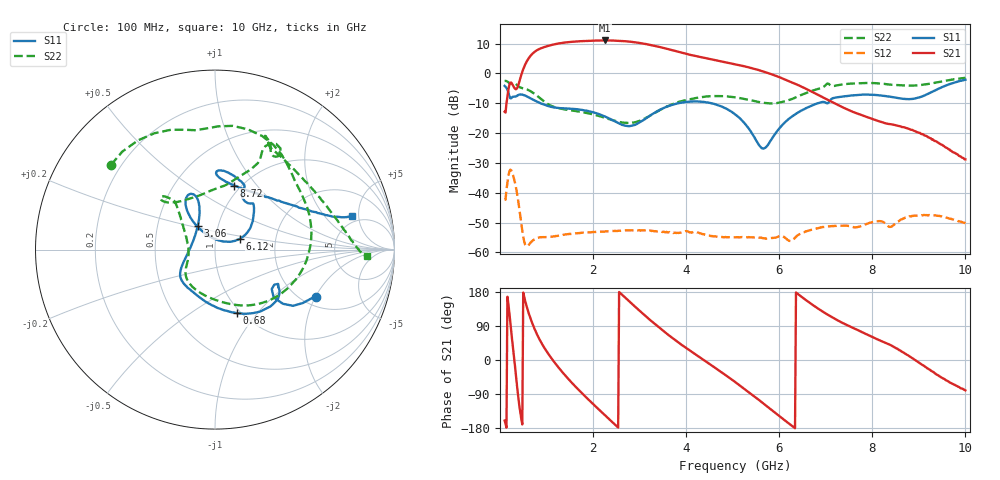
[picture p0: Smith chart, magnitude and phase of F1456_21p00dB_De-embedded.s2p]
! Integrated Device Technology
! Corporate Headquarters
! 6024 Silver Creek Valley Road
! San Jose, CA 95138  USA
! Phone:  1-408-284-8200
! Toll Free:  1-800-223-1366
! Webpage:  http://www.idt.com/
! Timing and RF Division
! 515 Groton Road, Suite 102
! Westford, MA 01886-6024
! Device:  F1456
! Description: 6-bit 0.5 dB Transmit Variable Gain Amplifier
! Frequency:  2100.0 -  2950.00 MHz
! Package:  6x6 mm Thin QFN Plastic Package: 28 pin
! State:  42
! Atten State:  21.0 dB
! Voltage:  +5.00 Volts
! Current:  216.984 mA
! Data:  The device was measured on a the F1455 evaluation board which has
!  individual transmission lines to the RF pins.  Data was collected
!  using a calibrated network analyzer.  The evaluation board was
!  de-embedded using a TRL calibration technique.
!  The reference plane is the edge of the package pin.
!  Pin  1 = CSb
!  Pin  2 = DATA
!  Pin  3 = CLK
!  Pin  4 = RSET
!  Pin  5 = GND
!  Pin  6 = RFIN  = Port 1
!  Pin  7 = GND
!  Pin  8 = NC
!  Pin  9 = NC
!  Pin 10 = NC
!  Pin 11 = NC
!  Pin 12 = NC
!  Pin 13 = NC
!  Pin 14 = /STBY
!  Pin 15 = GND
!  Pin 16 = RFOUT  = Port 2
!  Pin 17 = GND
!  Pin 18 = NC
!  Pin 19 = NC
!  Pin 20 = NC
!  Pin 21 = GND
!  Pin 22 = NC
!  Pin 23 = GND
!  Pin 24 = NC
!  Pin 25 = NC
!  Pin 26 = NC
!  Pin 27 = GND
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# GHz S dB R 50
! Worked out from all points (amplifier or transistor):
!   496 points, 100 MHz to 10 GHz, reference 50 ohm
!   highest |S21| = 11.1 dB at 2.26 GHz (marker M1)
!   |S21| within 3 dB of that: 826.6 MHz to 3.635 GHz (2.809 GHz wide, 126 % of centre)
!   unconditionally stable (mu >= 1): start of sweep to end of sweep
!   at 1.74 GHz: K = 60.34, MAG = 11.3 dB, |S12| = -53.5 dB
!   at 5.06 GHz: K = 157.94, MAG = 4.0 dB, |S12| = -54.9 dB
!   at 10 GHz: K = 490.62, MAG = -19.2 dB, |S12| = -50.2 dB
!   S11 on the Smith chart (normalised r, x): 100 MHz: 2.37, -2.01; 680 MHz: 0.96, -0.79; 3.06 GHz: 0.80, +0.21; 6.12 GHz: 1.31, +0.16; 8.72 GHz: 0.93, +0.77; 10 GHz: 4.20, +4.08
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0.1  -4.16 -25.0  -12.84 -160.0  -42.30 49.4  -2.53 140.8
0.22  -8.29 -34.8  -3.11 102.2  -32.25 -51.2  -3.44 99.1
0.3  -7.77 -30.5  -4.58 10.6  -35.17 -135.4  -3.16 74.8
0.42  -7.05 -37.4  -2.53 -124.1  -45.77 140.9  -4.60 41.1
0.54  -7.39 -54.0  2.92 156.8  -57.37 138.9  -5.14 15.7
0.68  -8.51 -70.7  6.33 101.5  -56.39 146.2  -6.17 -15.8
0.86  -9.89 -89.3  8.32 52.1  -54.96 113.1  -8.28 -52.0
1.16  -11.37 -114.3  9.74 -4.3  -54.65 76.5  -11.21 -92.5
1.48  -11.78 -131.7  10.53 -51.5  -53.85 52.3  -12.27 -119.8
1.76  -12.21 -142.0  10.84 -87.5  -53.42 36.2  -12.93 -134.4
2.26  -14.47 -158.1  11.07 -146.3  -52.98 12.5  -14.90 -151.3
2.64  -17.30 174.1  10.88 170.3  -52.71 -4.0  -16.47 -169.1
3.06  -15.85 126.7  10.07 123.4  -52.58 -23.9  -15.53 159.7
3.4  -12.49 111.3  8.99 87.6  -52.95 -39.3  -12.62 141.0
4.1  -9.40 113.4  6.20 23.4  -53.32 -70.3  -8.60 130.8
5.06  -13.78 128.0  3.09 -58.7  -54.94 -117.7  -8.03 137.1
5.66  -25.18 71.7  0.64 -114.7  -55.23 -155.9  -9.84 120.5
6.12  -16.42 23.6  -2.02 -159.3  -55.02 171.3  -9.29 87.6
6.7  -10.77 41.9  -6.12 147.0  -52.40 147.9  -5.86 64.9
8.36  -7.75 87.9  -16.95 41.4  -51.42 71.9  -3.72 62.4
8.72  -8.58 73.3  -18.28 15.9  -48.39 69.2  -4.02 50.2
10  -2.11 13.8  -28.80 -80.2  -50.23 -22.0  -1.46 -2.6
